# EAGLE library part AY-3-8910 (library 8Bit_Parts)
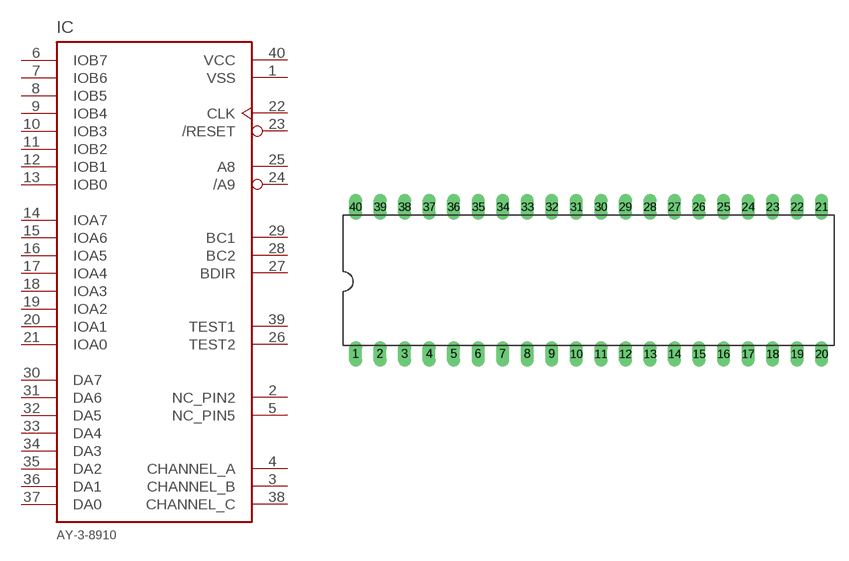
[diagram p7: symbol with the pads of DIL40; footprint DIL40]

Designator prefix IC

## AY-3-8910  [DIL40]
1  VSS  pwr
2  NC_PIN2  nc
3  CHANNEL_B  out
4  CHANNEL_A  out
5  NC_PIN5
6  IOB7
7  IOB6
8  IOB5
9  IOB4
10  IOB3
11  IOB2
12  IOB1
13  IOB0
14  IOA7
15  IOA6
16  IOA5
17  IOA4
18  IOA3
19  IOA2
20  IOA1
21  IOA0
22  CLK  in
23  /RESET  in
24  /A9
25  A8
26  TEST2  nc
27  BDIR  in
28  BC2  in
29  BC1  in
30  DA7
31  DA6
32  DA5
33  DA4
34  DA3
35  DA2
36  DA1
37  DA0
38  CHANNEL_C  out
39  TEST1  nc
40  VCC  pwr

## Footprint DIL40 (pad centres in mm)
Dual In Line Package
drill 0.813 long: 1 -24.13,-7.62; 2 -21.59,-7.62; 3 -19.05,-7.62; 4 -16.51,-7.62; 5 -13.97,-7.62; 6 -11.43,-7.62; 7 -8.89,-7.62; 8 -6.35,-7.62; 9 -3.81,-7.62; 10 -1.27,-7.62; 11 1.27,-7.62; 12 3.81,-7.62; 13 6.35,-7.62; 14 8.89,-7.62; 15 11.43,-7.62; 16 13.97,-7.62; 17 16.51,-7.62; 18 19.05,-7.62; 19 21.59,-7.62; 20 24.13,-7.62; 21 24.13,7.62; 22 21.59,7.62; 23 19.05,7.62; 24 16.51,7.62; 25 13.97,7.62; 26 11.43,7.62; 27 8.89,7.62; 28 6.35,7.62; 29 3.81,7.62; 30 1.27,7.62; 31 -1.27,7.62; 32 -3.81,7.62; 33 -6.35,7.62; 34 -8.89,7.62; 35 -11.43,7.62; 36 -13.97,7.62; 37 -16.51,7.62; 38 -19.05,7.62; 39 -21.59,7.62; 40 -24.13,7.62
